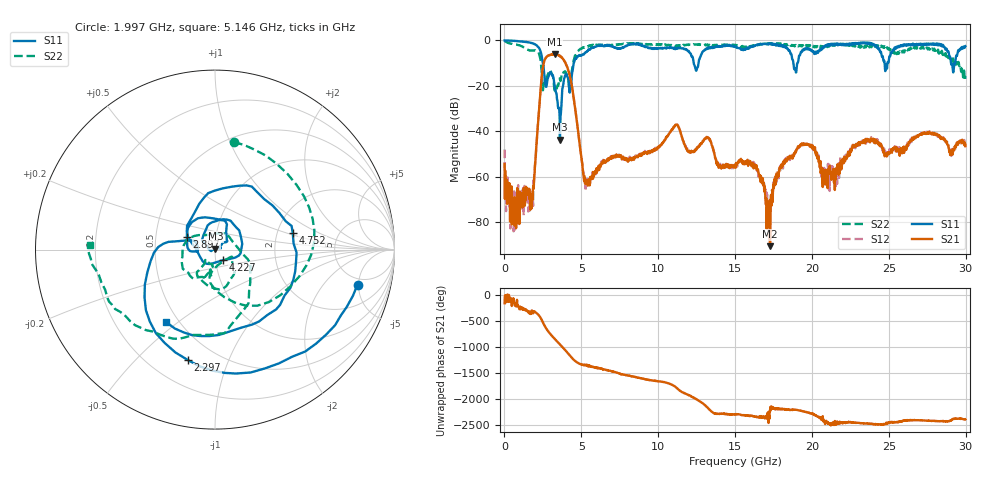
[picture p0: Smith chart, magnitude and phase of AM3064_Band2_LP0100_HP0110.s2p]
# Hz S DB R 50.0
!freq dBS11 angS11 dBS21 angS21 dBS12 angS12 dBS22 angS22
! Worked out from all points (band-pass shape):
!   1600 points, 10 MHz to 29.98 GHz, reference 50 ohm
!   highest |S21| = -6.00 dB at 3.271 GHz (marker M1); lowest = -90.4 dB at 17.27 GHz (marker M2)
!   |S21| within 3 dB of the highest: 2.595 GHz to 3.891 GHz (1.296 GHz wide, 40 % of centre)
!   lowest |S11| = -43.7 dB at 3.609 GHz (marker M3), VSWR 1.01, Z = 50.2 + j0.612 ohm
!   |S11| at or under -10 dB: 2.503 GHz to 4.508 GHz (2.005 GHz wide, 57.2 % of centre); 12.31 GHz to 12.62 GHz (308 MHz wide, 2.47 % of centre); 18.8 GHz to 19.05 GHz (252.4 MHz wide, 1.33 % of centre)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
!   |S22| runs from -22.1 to -0.3 dB; largest |S21 - S12| = 0.013
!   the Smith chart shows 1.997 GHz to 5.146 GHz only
!   S11 on the Smith chart (normalised r, x): 1.997 GHz: 4.10, -4.85; 2.297 GHz: 0.35, -0.72; 2.897 GHz: 0.72, +0.11; 4.227 GHz: 1.08, -0.13; 4.752 GHz: 2.44, +0.55; 5.146 GHz: 0.43, -0.45
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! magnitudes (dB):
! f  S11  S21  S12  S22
! 10 MHz  0.0  -54.3  -47.9  -0.3
! 534.8 MHz  -0.2  -71.1  -80.6  -1.5
! 1.716 GHz  -1.1  -74.0  -66.5  -4.5
! 1.997 GHz  -1.7  -54.5  -53.6  -4.3
! 2.297 GHz  -4.0  -26.1  -26.0  -7.0
! 2.897 GHz  -15.2  -6.5  -6.5  -13.4
! 3.271 GHz  -20.1  -6.0  -6.0  -22.1
! 3.609 GHz  -43.7  -6.9  -6.8  -17.1
! 4.227 GHz  -22.7  -15.0  -14.9  -20.8
! 4.752 GHz  -7.1  -37.9  -37.9  -5.1
! 5.015 GHz  -6.7  -52.0  -51.7  -3.6
! 5.146 GHz  -6.3  -59.4  -58.1  -3.1
! 10 GHz  -3.5  -46.9  -46.9  -1.8
! 11.2 GHz  -3.6  -37.2  -37.1  -2.4
! 15 GHz  -2.7  -54.7  -54.7  -2.0
! 16.34 GHz  -2.2  -55.0  -55.5  -2.4
! 17.27 GHz  -1.5  -90.4  -75.9  -1.3
! 18.15 GHz  -2.8  -53.9  -53.1  -2.0
! 19.99 GHz  -4.3  -46.3  -47.3  -2.2
! 20.85 GHz  -2.7  -56.9  -62.8  -2.9
! 25 GHz  -9.1  -49.1  -49.1  -3.4
! 29.98 GHz  -2.5  -46.5  -45.6  -15.8
